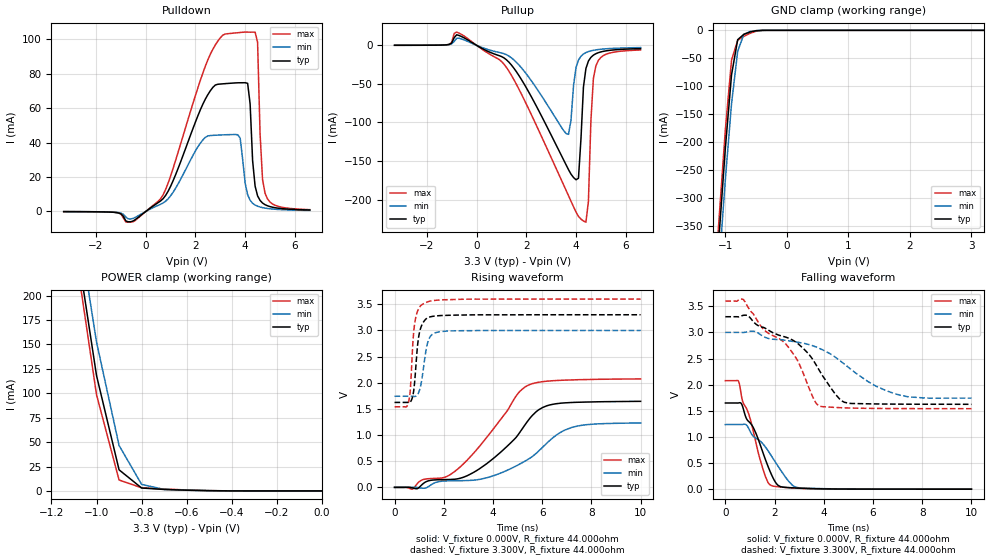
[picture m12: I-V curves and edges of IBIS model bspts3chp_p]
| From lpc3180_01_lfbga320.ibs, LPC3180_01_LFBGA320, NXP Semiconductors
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| |   Rev 0.20 IBIS Model Design Automation Generation   |
| |   N O N - S I L I C O N   C O R R E L A T E D   |
| |   This IBIS [Model] is pre-Beta tactical support   |
| |  Note: this IBIS [Model] contains clamp curves generated   |
| |   through simulation which should not be relied upon   |
| bspts3chp
|   Bidirectional Pad 3v3
|   3state Output
|   Plain Input
|   3ns Slew Rate control
|   CMOS
|   Programmable between
|   - (p1=0, p2=1) plain input
|   - (p1=0, p2=0) with Pull Up
|   - (p1=1, p2=1) with Pull Down
|   - (p1=1, p2=0) with Repeater
|   Characterized at Core 1.2V and I/O 3.3V
| Plain input Mode (p1=0, p2=1)
[Model]   bspts3chp_p | of bspts3chp
Model_type   I/O
Polarity   Non-Inverting
Enable   Active-Low
|  Reciever Thresholds
Vinl   = 0.36V
Vinh   = 0.84V
| AC Test Load Conditions
Vref   = 0
Cref   = 1.2e-11
Rref   = 1000000000
Vmeas   = 0.6
| [Process Range]   typical   min   max
| C_comp edge width   400.000ps   400.000ps   400.000ps
| C_comp Tstrobe   40.000fs   40.000fs   40.000fs
C_comp   2.386pF   2.238pF   2.565pF
[Temperature Range]   25   125   -40
[Voltage Range]   3.30V   3.00V   3.60V
[GND Clamp Reference]   0.00V   0.00V   0.00V
[Pulldown Reference]   0.00V   0.00V   0.00V
[POWER Clamp Reference]   3.30V   3.00V   3.60V
[Pullup Reference]   3.30V   3.00V   3.60V
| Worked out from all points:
|   slope of the pulldown table from 0 to 0.495 V, typ, clamps not added: 97.1 ohm
|   slope of the pullup table from 0 to 0.495 V, typ, clamps not added: 59.3 ohm
|   GND clamp passes 1 mA (typ) near -0.51 V on its own axis
|   POWER clamp passes 1 mA (typ) near -0.63 V on its own axis
|   rising waveform, V_fixture 0.000V, R_fixture 44.000ohm: 20-80 % time 2.13ns typ, 2.37ns min, 2.1ns max; typ from 0 V to 1.65 V
|   falling waveform, V_fixture 0.000V, R_fixture 44.000ohm: 20-80 % time 928ps typ, 1.23ns min, 792ps max; typ from 1.65 V to 0 V
|   rising waveform, V_fixture 3.300V, R_fixture 44.000ohm: 20-80 % time 211ps typ, 252ps min, 185ps max; typ from 1.62 V to 3.3 V
|   falling waveform, V_fixture 3.300V, R_fixture 44.000ohm: 20-80 % time 2.17ns typ, 2.52ns min, 2.04ns max; typ from 3.3 V to 1.62 V
[GND Clamp]
| ref voltage   0.00V   0.00V   0.00V
|   Voltage   I(typ)   I(min)   I(max)
-3.3V     -4.198A    -4.223A    -4.188A
-1.2V     -526mA     -577.5mA   -497.2mA
-1.1V     -363.6mA   -417.9mA   -332.6mA
-1V       -210.1mA   -266.3mA   -177.3mA
-900mV    -79.7mA    -131.5mA   -53.27mA
-800mV    -16.73mA   -37.37mA   -17.76mA
-700mV    -7.134mA   -7.247mA   -10.88mA
-600mV    -2.975mA   -2.186mA   -5.408mA
-500mV    -676.3uA   -558.4uA   -1.581mA
-400mV    -60.83uA   -85.23uA   -138.3uA
3.2V      712.7pA    549nA      572.1pA
[Power Clamp]   | Vtable = Vcc - Vpad
| ref voltage   3.30V   3.00V   3.60V
|   Voltage   I(typ)   I(min)   I(max)
-3.3V     4.52A      4.504A     4.537A
-1.1V     269.9mA    299.6mA    255.3mA
-1V       118.1mA    152.4mA    98.46mA
-900mV    21.59mA    46.52mA    11.18mA
-800mV    2.991mA    6.661mA    3.207mA
-700mV    1.495mA    1.535mA    1.933mA
-600mV    740.8uA    686.9uA    976.4uA
-400mV    40.41uA    69.77uA    40.29uA
0V        755pA      5.591nA    627.8pA
[Pulldown]
| ref voltage   0.00V   0.00V   0.00V
|   Voltage   I(typ)   I(min)   I(max)
-3.3V     -80.68uA   -69.9uA    -74.32uA
-600mV    -5.92mA    -4.329mA   -6.173mA
500mV     5.147mA    3.568mA    5.923mA
2.5V      67.8mA     43.83mA    87.99mA
3.7V      74.65mA    44.53mA    103.7mA
4V        74.69mA    16.44mA    104.1mA
4.2V      62.37mA    6.515mA    104mA
4.3V      29.48mA    4.769mA    104mA
4.5V      9.068mA    3.068mA    98.16mA
4.6V      6.413mA    2.587mA    45.13mA
4.8V      3.956mA    1.96mA     10.6mA
6.6V      844.8uA    597.5uA    1.056mA
[Pullup]   | Vtable = Vcc - Vpad
| ref voltage   3.30V   3.00V   3.60V
|   Voltage   I(typ)   I(min)   I(max)
-3.3V     39.4uA     37.84uA    38.83uA
-800mV    13.66mA    9.122mA    17.15mA
1V        -14.52mA   -9.936mA   -20.86mA
3.7V      -161.3mA   -115.5mA   -195.1mA
4V        -174.4mA   -29.02mA   -216.2mA
4.1V      -172.4mA   -19.17mA   -221.9mA
4.4V      -30.01mA   -9.422mA   -229.4mA
4.5V      -20.39mA   -8.135mA   -202.5mA
4.6V      -15.6mA    -7.195mA   -97.89mA
4.7V      -12.75mA   -6.48mA    -42.98mA
4.8V      -10.87mA   -5.92mA    -26.67mA
6.6V      -4.278mA   -2.929mA   -6.056mA
[Ramp]
R_load   = 44.000ohm
|   dV/dt(typ)   dV/dt(min)   dV/dt(max)
dV/dt_r   1.000V/2.135ns   750.815mV/2.380ns   1.259V/2.105ns
dV/dt_f   1.022V/2.190ns   769.258mV/2.465ns   1.253V/2.030ns
[Rising Waveform]  | cubic spline decimation from 2001 points
V_fixture   = 0.000V
R_fixture   = 44.000ohm
|   Time   V(typ)   V(min)   V(max)
0s        20.67nV    394.6nV    10.71nV
730ps     -10.43mV   1.454mV    -33.2mV
1.11ns    49.31mV    -14.32mV   140mV
2.455ns   156.3mV    126.9mV    306.7mV
4.055ns   567.9mV    227.8mV    1.141V
5.025ns   1.008V     429.7mV    1.799V
5.5ns     1.321V     557.4mV    1.967V
6.185ns   1.559V     843.2mV    2.03V
7.21ns    1.623V     1.147V     2.054V
10ns      1.645V     1.231V     2.073V
[Falling Waveform]  | cubic spline decimation from 2001 points
V_fixture   = 0.000V
R_fixture   = 44.000ohm
|   Time   V(typ)   V(min)   V(max)
0s        1.649V     1.237V     2.077V
535ps     1.65V      1.237V     2.064V
695ps     1.59V      1.238V     1.692V
845ps     1.362V     1.232V     1.556V
1.16ns    1.155V     998.9mV    1.058V
1.565ns   648.7mV    845.2mV    330.1mV
1.89ns    261.6mV    622.8mV    65.34mV
2.22ns    52.62mV    382.7mV    42.94mV
2.94ns    20.57mV    29.77mV    17.37mV
10ns      25.57uV    53.57uV    21.14uV
[Rising Waveform]  | cubic spline decimation from 2001 points
V_fixture   = 3.300V
V_fixture_min = 3.000V
V_fixture_max = 3.600V
R_fixture   = 44.000ohm
|   Time   V(typ)   V(min)   V(max)
0s        1.624V     1.742V     1.54V
535ps     1.623V     1.743V     1.58V
625ps     1.626V     1.743V     1.785V
700ps     1.683V     1.742V     2.364V
780ps     1.851V     1.739V     2.977V
865ps     2.302V     1.743V     3.254V
1.025ns   2.983V     1.875V     3.451V
1.32ns    3.234V     2.721V     3.542V
2.17ns    3.289V     2.989V     3.588V
10ns      3.3V       3V         3.6V
[Falling Waveform]  | cubic spline decimation from 2001 points
V_fixture   = 3.300V
V_fixture_min = 3.000V
V_fixture_max = 3.600V
R_fixture   = 44.000ohm
|   Time   V(typ)   V(min)   V(max)
0s        3.3V       3V         3.6V
735ps     3.327V     2.998V     3.627V
1.515ns   3.099V     2.93V      3.078V
2.435ns   2.912V     2.849V     2.788V
3.2ns     2.677V     2.789V     2.176V
3.855ns   2.243V     2.687V     1.586V
4.635ns   1.729V     2.468V     1.56V
5.04ns    1.642V     2.317V     1.553V
7.13ns    1.627V     1.795V     1.542V
10ns      1.624V     1.742V     1.54V
